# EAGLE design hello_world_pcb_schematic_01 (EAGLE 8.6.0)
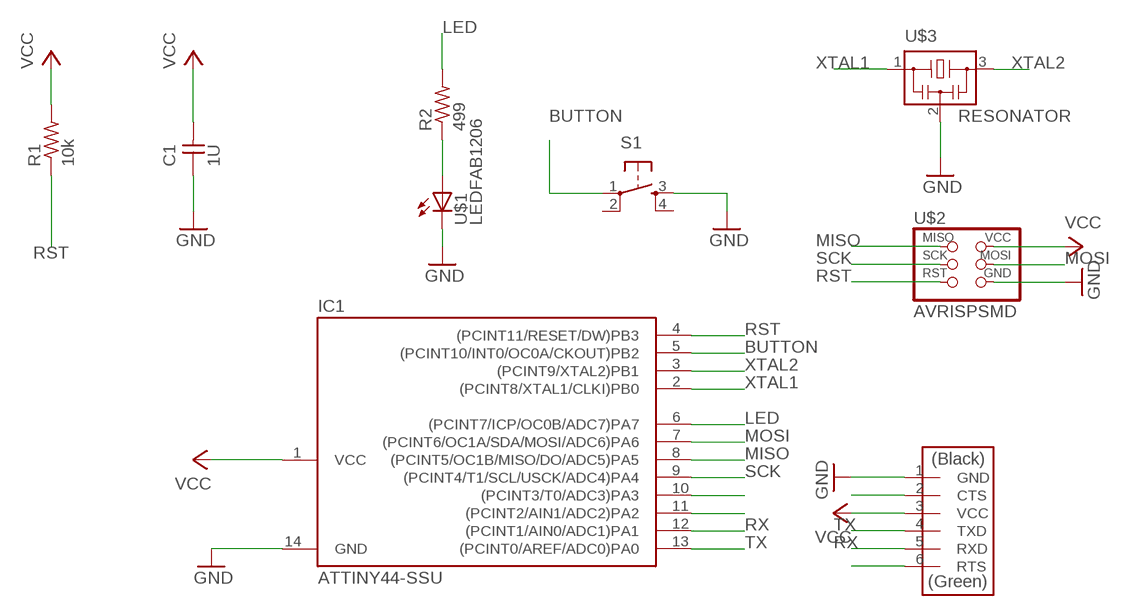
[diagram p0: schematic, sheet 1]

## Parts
C1  1U  CAP-UNPOLARIZEDFAB  [C1206FAB]
IC1  ATTINY44-SSU  [SOIC14]
R1  10k  RES-US1206FAB  [R1206FAB]
R2  499  RES-US1206FAB  [R1206FAB]
S1  6MM_SWITCH6MM_SWITCH  [6MM_SWITCH]
U$1  LEDFAB1206  [LED1206FAB]
U$2  AVRISPSMD  [2X03SMD]
U$3  RESONATOR  [EFOBM]
U$4  FTDI-SMD-HEADER  [1X06SMD]

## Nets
BUTTON: IC1.5((PCINT10/INT0/OC0A/CKOUT)PB2) S1.1(P)
GND: C1.1 IC1.14(GND) S1.3(S) U$1.2(C) U$2.6(GND) U$3.2 U$4.1(GND)
LED: IC1.6((PCINT7/ICP/OC0B/ADC7)PA7) R2.2
MISO: IC1.8((PCINT5/OC1B/MISO/DO/ADC5)PA5) U$2.1(MISO)
MOSI: IC1.7((PCINT6/OC1A/SDA/MOSI/ADC6)PA6) U$2.4(MOSI)
N$1: R2.1 U$1.1(A)
N$9: IC1.10((PCINT3/T0/ADC3)PA3)
N$10: IC1.11((PCINT2/AIN1/ADC2)PA2)
N$23: U$4.2(CTS)
N$27: U$4.6(RTS)
RST: IC1.4((PCINT11/RESET/DW)PB3) R1.1 U$2.5(RST)
RX: IC1.12((PCINT1/AIN0/ADC1)PA1) U$4.5(RXD)
SCK: IC1.9((PCINT4/T1/SCL/USCK/ADC4)PA4) U$2.3(SCK)
TX: IC1.13((PCINT0/AREF/ADC0)PA0) U$4.4(TXD)
VCC: C1.2 IC1.1(VCC) R1.2 U$2.2(VCC) U$4.3(VCC)
XTAL1: IC1.2((PCINT8/XTAL1/CLKI)PB0) U$3.1
XTAL2: IC1.3((PCINT9/XTAL2)PB1) U$3.3
Unconnected: S1.2(P1) S1.4(S1)

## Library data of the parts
C1 = fab:CAP-UNPOLARIZED
IC1 = fab:ATTINY44
R1 R2 = fab:RES-US: Resistor (US Symbol)
S1 = fab:6MM_SWITCH: OMRON SWITCH
U$1 = fab:LED: LED
U$2 = fab:AVRISP
U$3 = fab:RESONATOR
U$4 = fab:FTDI-SMD-HEADER

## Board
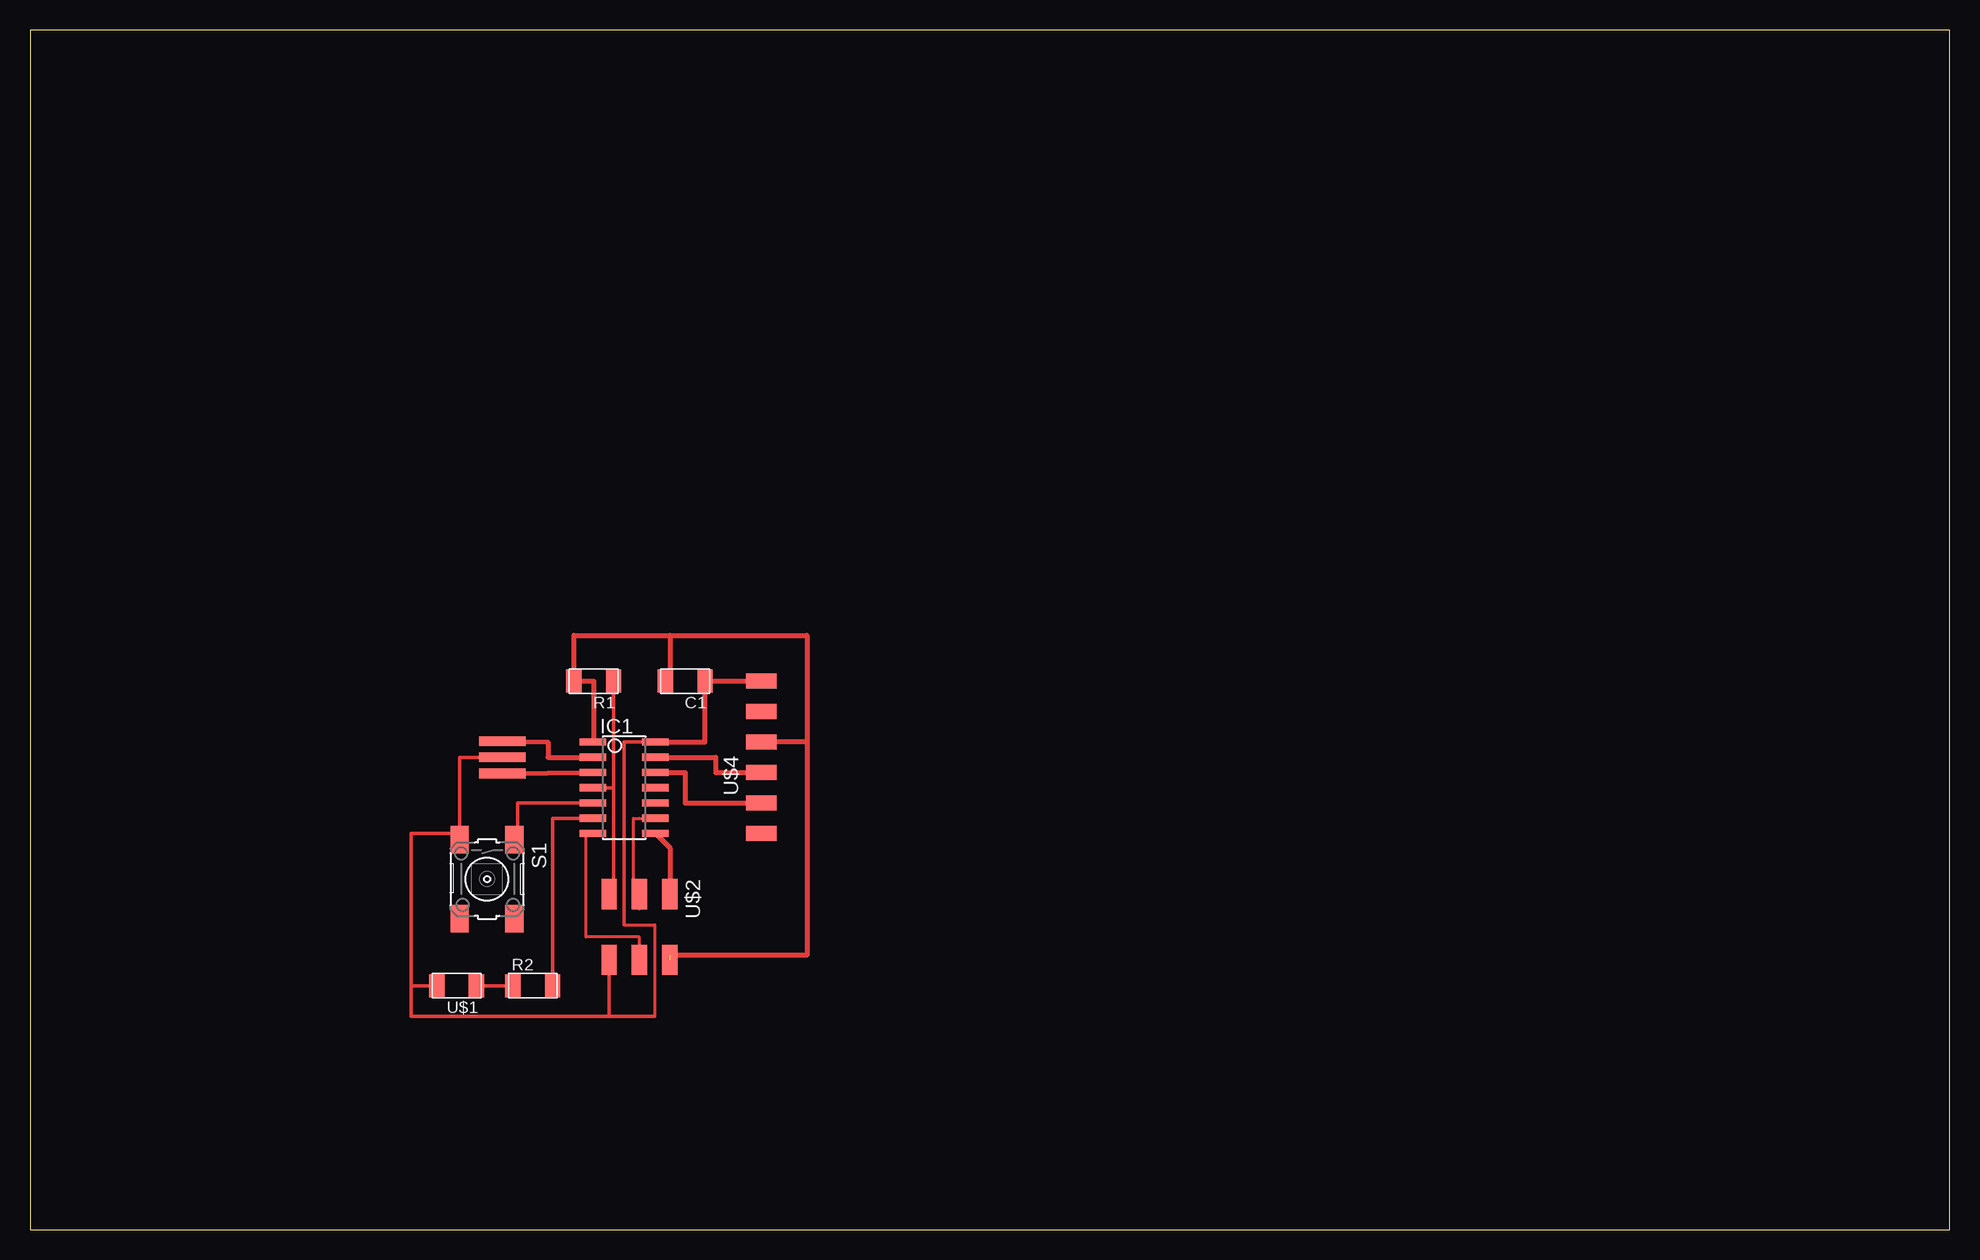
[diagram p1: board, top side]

Size 160 x 100 mm. Coordinates in mm from the lower left corner, seen from the top.
Outline: 0,0 160,0 160,100 0,100 0,0
Copper layers (1*16): Top 0.035mm / dielectric 1.5mm / Bottom 0.035mm
Design rules "default *": minimum track width 6mil, minimum drill 0.35mm, track to track 16mil, track to pad 16mil, pad to pad 16mil, via to via 16mil, smd to smd 16mil, copper to edge 40mil, drill to drill 6mil, minimum pad ring 10mil, minimum via ring 8mil, stop-mask expansion 4mil, vias tented up to drill 0mil, thermal gap 10mil

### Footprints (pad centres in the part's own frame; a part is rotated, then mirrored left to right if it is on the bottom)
C1206FAB = smd 1.27 x 1.905: 1 -1.651,0; 2 1.651,0
SOIC14 = smd 0.61 x 2.21: 1 -3.81,-2.603; 2 -2.54,-2.603; 3 -1.27,-2.603; 4 0,-2.603; 5 1.27,-2.603; 6 2.54,-2.603; 7 3.81,-2.603; 8 3.81,2.603; 9 2.54,2.603; 10 1.27,2.603; 11 0,2.603; 12 -1.27,2.603; 13 -2.54,2.603; 14 -3.81,2.603
R1206FAB = smd 1.27 x 1.905: 1 -1.651,0; 2 1.651,0
6MM_SWITCH = smd 2.286 x 1.524: 1 -3.302,2.286; 2 3.302,2.286; 3 -3.302,-2.286; 4 3.302,-2.286
LED1206FAB = smd 1.27 x 1.905: 1 -1.651,0; 2 1.651,0
2X03SMD = smd 2.54 x 1.27: 1 -2.54,2.54; 2 2.92,2.54; 3 -2.54,0; 4 2.92,0; 5 -2.54,-2.54; 6 2.92,-2.54
EFOBM = smd 0.8 x 3.9: 1 -1.35,0; 2 0,0; 3 1.35,0
1X06SMD = smd 2.54 x 1.27: 1 0,6.35; 2 0,3.81; 3 0,1.27; 4 0,-1.27; 5 0,-3.81; 6 0,-6.35

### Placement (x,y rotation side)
C1  54.61,45.72 180 top
IC1  49.53,36.83 270 top
R1  46.99,45.72 180 top
R2  41.91,20.32 0 top
S1  38.1,29.21 270 top
U$1  35.56,20.32 180 top
U$2  50.8,25.4 270 top
U$3  39.37,39.37 270 top
U$4  60.96,39.37 0 top

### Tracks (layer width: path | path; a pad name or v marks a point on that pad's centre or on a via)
BUTTON
  Top 0.305: IC1.5 40.64,35.56 40.64,32.51 S1.1
GND
  Top 0.152: 53.72,40.64 IC1.14
  Top 0.254: 52.07,17.78 52.07,25.4 49.53,25.4
  Top 0.305: IC1.14 49.53,40.64 49.53,25.4 | 52.07,17.78 48.26,17.78 | 48.26,17.78 U$2.6 | 48.26,17.78 31.75,17.78 31.75,20.32 | 31.75,20.32 U$1.2 | 31.75,20.32 31.75,33.02 35.56,33.02 35.56,32.51 S1.3 35.81,39.37 U$3.2
  Top 0.406: IC1.14 56.26,40.64 C1.1 U$4.1
LED
  Top 0.305: R2.2 43.56,34.29 IC1.6
MISO
  Top 0.406: IC1.8 53.34,31.81 U$2.1
MOSI
  Top 0.254: U$2.4 50.8,24.38 46.33,24.38 46.33,32.92 IC1.7
N$1
  Top 0.305: R2.1 U$1.1
RST
  Top 0.305: R1.1 48.64,36.83 | 48.64,36.83 IC1.4 | 48.64,36.83 48.64,27.94 U$2.5
RX
  Top 0.406: IC1.12 54.61,38.1 54.61,35.56 U$4.5
SCK
  Top 0.152: 50.8,26.67 U$2.3
  Top 0.254: IC1.9 50.8,34.29 50.29,34.29 50.29,27.94 U$2.3
TX
  Top 0.406: IC1.13 57.15,39.37 57.15,38.1 U$4.4
VCC  (2 unrouted)
  Top 0.406: 53.34,49.53 53.34,45.72 C1.2 | 53.34,49.53 45.34,49.53 R1.2 46.99,45.72 46.99,40.64 | 53.34,49.53 64.77,49.53 64.77,40.64 | 64.77,40.64 U$4.3 | 64.77,40.64 64.77,22.86 53.34,22.86
XTAL1
  Top 0.152: U$3.1 39.37,40.64
  Top 0.406: U$3.1 43.18,40.64 43.18,39.37 IC1.2
XTAL2
  Top 0.152: 46.93,38.02 IC1.3
  Top 0.406: U$3.3 IC1.3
